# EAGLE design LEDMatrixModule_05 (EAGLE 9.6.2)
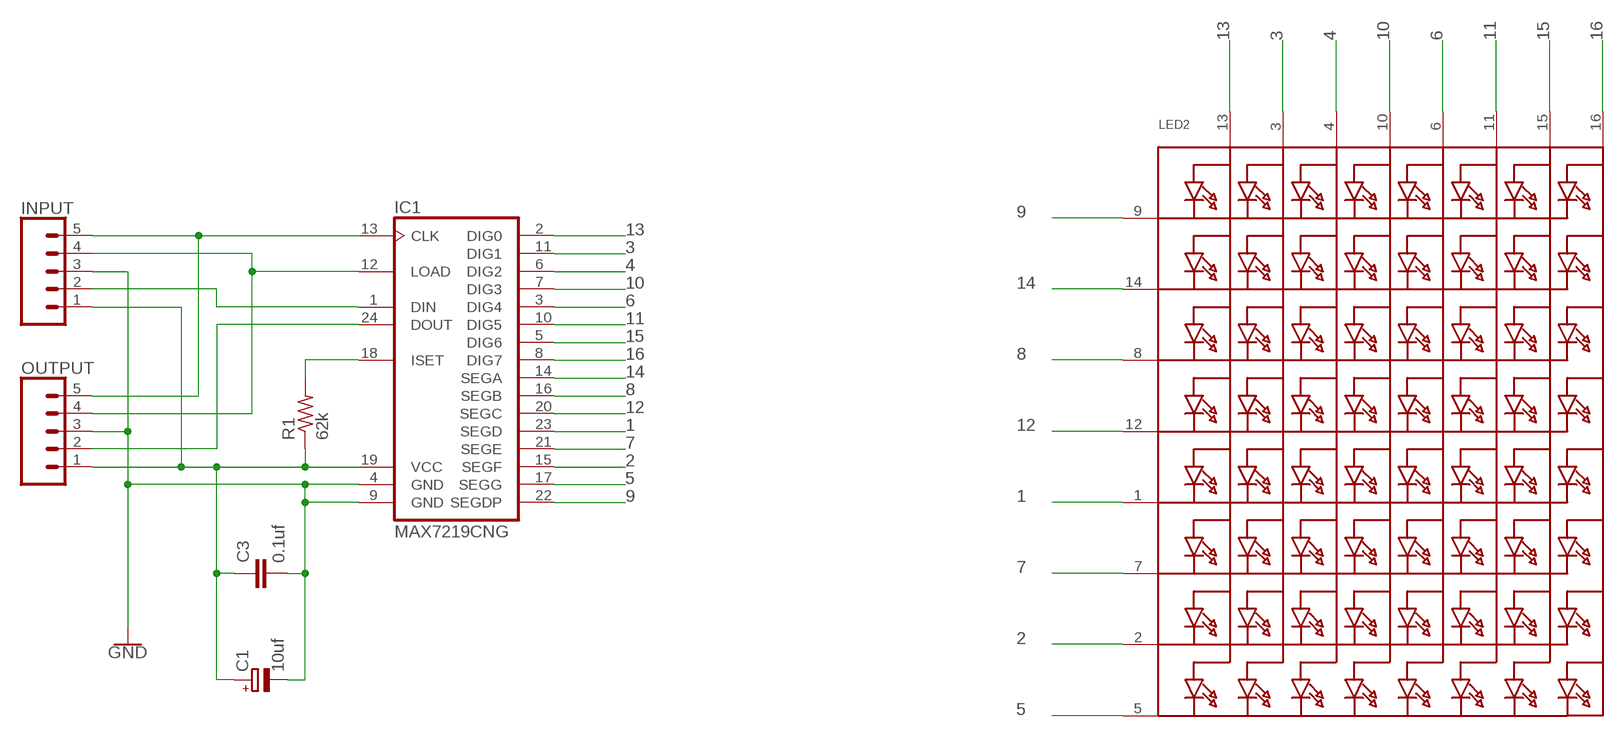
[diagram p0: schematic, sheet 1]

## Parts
C1  10uf  CPOL-EUE2.5-6  [E2,5-6]
C3  0.1uf  C2,5-3  [C2.5-3]
IC1  MAX7219CNG  [DIL24-3]
INPUT  CONN_05  [1X05]
LED2  SEGMENT_8X8_ROWCATHODEBL-M15  [SEGMENT_BL-M15A881]
OUTPUT  CONN_05  [1X05]
R1  62k  R-US_0309/10  [0309/10]

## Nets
1: IC1.23(SEGD) LED2.1(K5)
2: IC1.15(SEGF) LED2.2(K7)
3: IC1.11(DIG1) LED2.3(A2)
4: IC1.6(DIG2) LED2.4(A3)
5: IC1.17(SEGG) LED2.5(K8)
6: IC1.3(DIG4) LED2.6(A5)
7: IC1.21(SEGE) LED2.7(K6)
8: IC1.16(SEGB) LED2.8(K3)
9: IC1.22(SEGDP) LED2.9(K1)
10: IC1.7(DIG3) LED2.10(A4)
11: IC1.10(DIG5) LED2.11(A6)
12: IC1.20(SEGC) LED2.12(K4)
13: IC1.2(DIG0) LED2.13(A1)
14: IC1.14(SEGA) LED2.14(K2)
15: IC1.5(DIG6) LED2.15(A7)
16: IC1.8(DIG7) LED2.16(A8)
GND: C1.- C3.2 IC1.4(GND) IC1.9(GND) INPUT.3 OUTPUT.3
N$1: IC1.13(CLK) INPUT.5 OUTPUT.5
N$2: C1.+ C3.1 IC1.19(VCC) INPUT.1 OUTPUT.1 R1.1
N$3: IC1.18(ISET) R1.2
N$4: IC1.24(DOUT) OUTPUT.2
N$5: IC1.1(DIN) INPUT.2
N$6: IC1.12(LOAD) INPUT.4 OUTPUT.4

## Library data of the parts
C1 = rcl:CPOL-EU: POLARIZED CAPACITOR, European symbol
C3 = capacitor-wima:C: CAPACITOR
IC1 = max7219:MAX7219CNG: LED DISPLAY DRIVER; MF: MAXIM; MPN: MAX7219CNG; OC_FARNELL: 1523914; OC_NEWARK: 34C4018
INPUT OUTPUT = SparkFun-Connectors:CONN_05: Multi connection point. Often used as Generic Header-pin footprint for 0.1 inch spaced/style header connections On any of the 0.1 inch spaced packages, you can populate with these: Break Away Headers - Straight (PRT-00116) Break Away Male Headers - Right Angle (PRT-00553) Female Headers (PRT-00115)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
LED2 = adafruit:SEGMENT_8X8_ROWCATHODE: 8x8 LED Segment Displays: Row = Cathode 0.7" Red 8X8 Matrix, 1.9mm Round LEDs - BL-M07C881UR 1.2" Red 8x8 Matrix, 3.0mm Round LEDs - BL-M12A881UR 1.2" Red 8x8 Matrix, 3.0mm Square LEDs - BL-M12A883
R1 = BeagleBone_Black_Wireless:R-US_: RESISTOR, American symbol

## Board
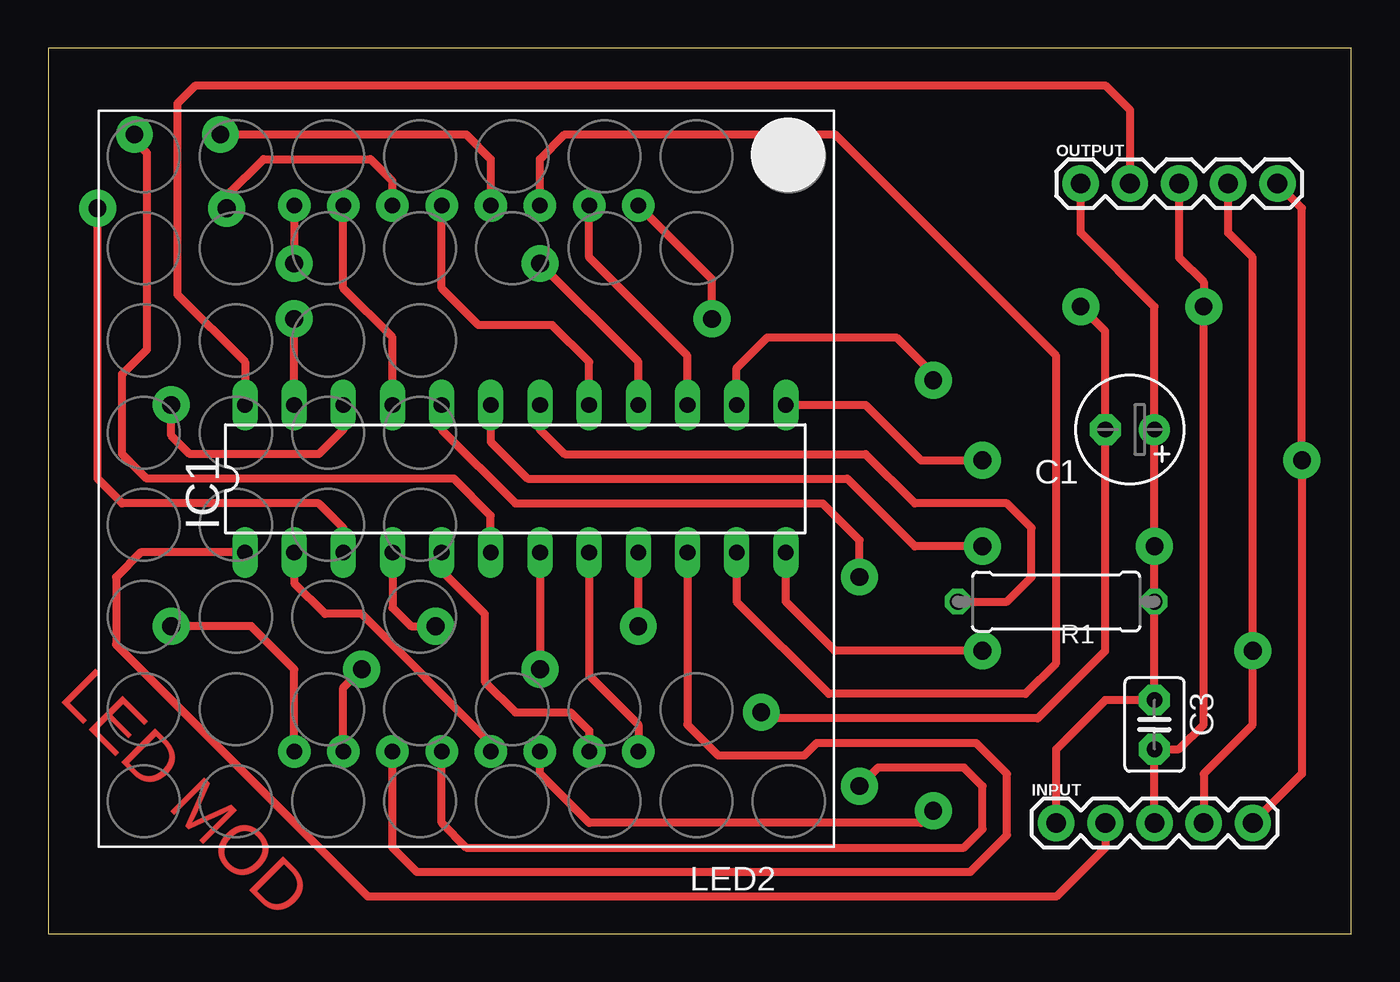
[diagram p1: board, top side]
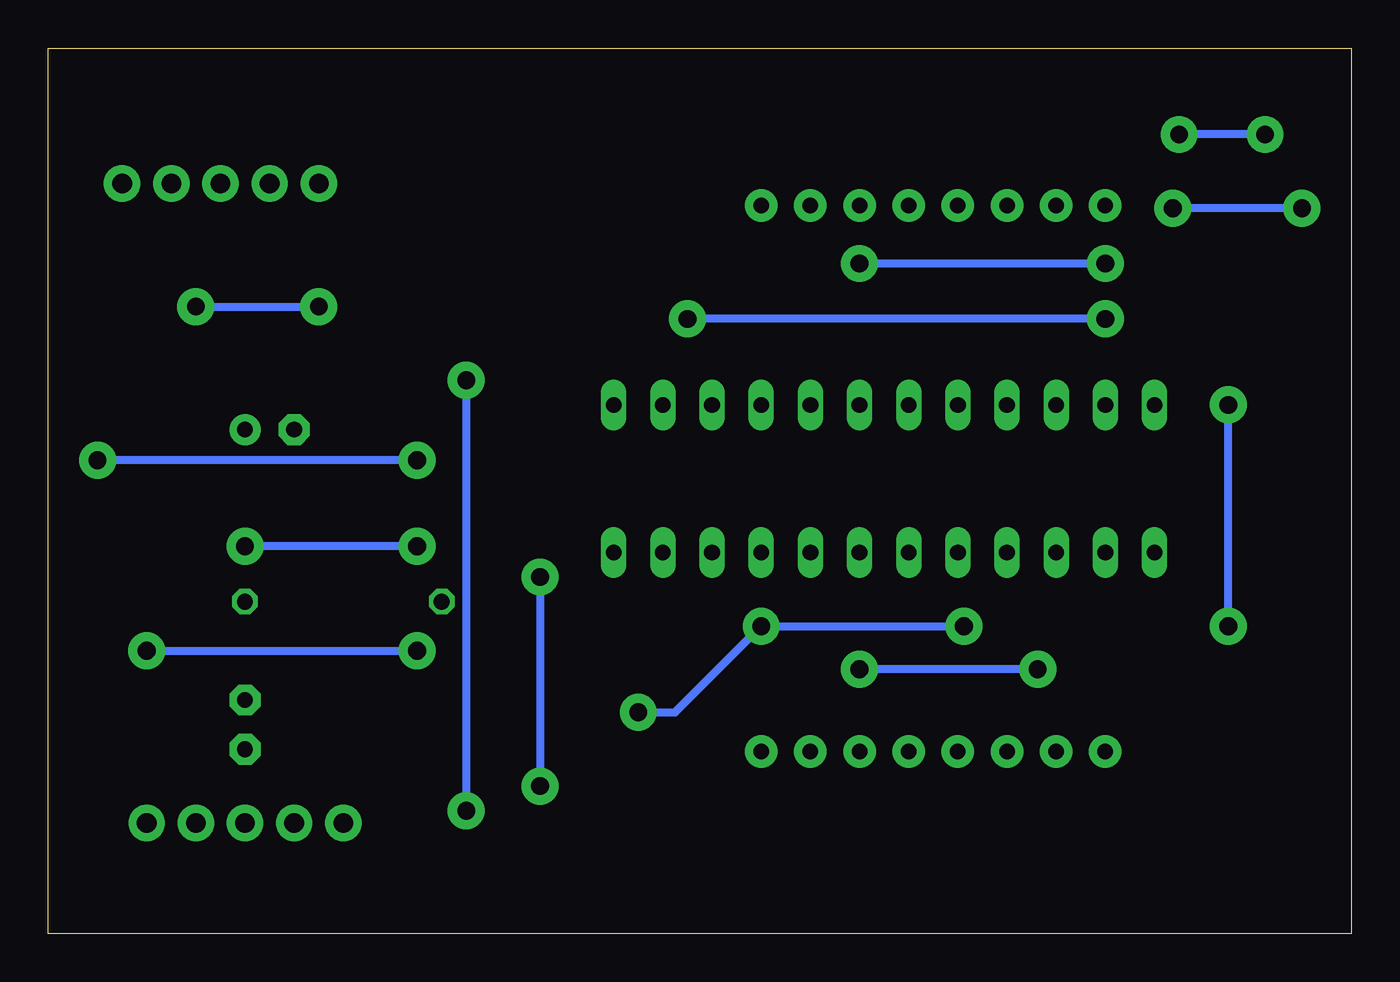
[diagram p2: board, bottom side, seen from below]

Size 67.31 x 45.72 mm. Coordinates in mm from the lower left corner, seen from the top.
Outline: 0,0 67.31,0 67.31,45.72 0,45.72 0,0
Copper layers (1*16): Top 0.035mm / dielectric 1.5mm / Bottom 0.035mm
Design rules "default": minimum track width 10mil, minimum drill 24mil, track to track 8mil, track to pad 8mil, pad to pad 8mil, via to via 8mil, smd to smd 8mil, copper to edge 40mil, drill to drill 8mil, minimum pad ring 10mil, minimum via ring 8mil, stop-mask expansion 4mil, vias tented up to drill 0mil, thermal gap 10mil

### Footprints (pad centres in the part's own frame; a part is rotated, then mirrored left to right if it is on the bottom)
E2,5-6 = drill 0.813 pad 1.6: + -1.27,0 | drill 0.813 pad 1.6 octagon: - 1.27,0
C2.5-3 = drill 0.813 pad 1.6 octagon: 1 -1.27,0; 2 1.27,0
DIL24-3 = drill 0.813 long: 1 -13.97,-3.81; 2 -11.43,-3.81; 3 -8.89,-3.81; 4 -6.35,-3.81; 5 -3.81,-3.81; 6 -1.27,-3.81; 7 1.27,-3.81; 8 3.81,-3.81; 9 6.35,-3.81; 10 8.89,-3.81; 11 11.43,-3.81; 12 13.97,-3.81; 13 13.97,3.81; 14 11.43,3.81; 15 8.89,3.81; 16 6.35,3.81; 17 3.81,3.81; 18 1.27,3.81; 19 -1.27,3.81; 20 -3.81,3.81; 21 -6.35,3.81; 22 -8.89,3.81; 23 -11.43,3.81; 24 -13.97,3.81
1X05 = drill 1.016 pad 1.88: 1 0,0; 2 2.54,0; 3 5.08,0; 4 7.62,0; 5 10.16,0
SEGMENT_BL-M15A881 = drill 0.8 pad 1.676: 1 -8.89,-14.1; 2 -6.35,-14.1; 3 -3.81,-14.1; 4 -1.27,-14.1; 5 1.27,-14.1; 6 3.81,-14.1; 7 6.35,-14.1; 8 8.89,-14.1; 9 8.89,14.1; 10 6.35,14.1; 11 3.81,14.1; 12 1.27,14.1; 13 -1.27,14.1; 14 -3.81,14.1; 15 -6.35,14.1; 16 -8.89,14.1
0309/10 = drill 0.813 octagon: 1 -5.08,0; 2 5.08,0

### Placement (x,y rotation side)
C1  55.88,26.04 180 top
C3  57.15,10.79 270 top
IC1  24.13,23.5 0 top
INPUT  52.07,5.71 0 top
LED2  21.59,23.5 180 top
OUTPUT  53.34,38.73 0 top
R1  52.07,17.14 180 top

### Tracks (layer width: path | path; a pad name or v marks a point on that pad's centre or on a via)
1  (via drill 0.91 pad 1.91)
  Top 0.406: IC1.23 v12.7,31.75 | v34.29,31.75 34.29,33.78 LED2.1
  Bottom 0.406: v12.7,31.75 v34.29,31.75
2
  Top 0.406: IC1.15 33.02,29.84 27.94,34.92 LED2.2
3
  Top 0.406: IC1.11 35.56,17.14 40.32,12.38 50.48,12.38 52.07,13.97 52.07,29.84 40.64,41.27 26.67,41.27 25.4,40.01 LED2.3
4  (via drill 0.91 pad 1.91)
  Top 0.406: v8.89,41.27 21.59,41.27 22.86,40.01 LED2.4 | v4.45,41.27 4.45,40.96 5.08,40.32 5.08,30.16 3.81,28.89 3.81,24.77 5.08,23.5 20.95,23.5 22.86,21.59 IC1.6
  Bottom 0.406: v4.45,41.27 v8.89,41.27
5
  Top 0.406: IC1.17 27.94,29.53 26.04,31.43 22.23,31.43 20.32,33.34 LED2.5
6  (via drill 0.91 pad 1.91)
  Top 0.406: IC1.3 15.24,20.95 13.97,22.23 3.81,22.23 2.54,23.5 v2.54,37.47 | LED2.6 17.78,38.87 16.64,40.01 11.11,40.01 9.21,38.1 v9.21,37.47
  Bottom 0.406: v2.54,37.47 v9.21,37.47
7
  Top 0.406: IC1.21 17.78,30.8 15.24,33.34 LED2.7
8  (via drill 0.91 pad 1.91)
  Top 0.406: IC1.16 30.48,29.53 v25.4,34.61 | LED2.8 v12.7,34.61
  Bottom 0.406: v12.7,34.61 v25.4,34.61
9  (via drill 0.91 pad 1.91)
  Top 0.406: IC1.22 15.24,26.04 13.97,24.77 7.3,24.77 6.35,25.72 v6.35,27.3 | LED2.9 12.7,13.65 10.48,15.88 v6.35,15.88
  Bottom 0.406: v6.35,15.88 v6.35,27.3
10  (via drill 0.91 pad 1.91)
  Top 0.406: IC1.7 v25.4,13.65 | LED2.10 15.24,12.7 v16.19,13.65
  Bottom 0.406: v16.19,13.65 v25.4,13.65
11
  Top 0.406: LED2.11 17.78,4.45 19.05,3.17 47.62,3.17 49.53,5.08 49.53,8.26 47.94,9.84 39.69,9.84 39.05,9.21 34.61,9.21 33.02,10.79 IC1.10
12  (via drill 0.91 pad 1.91)
  Top 0.406: LED2.12 20.32,5.71 21.59,4.45 47.31,4.45 48.26,5.4 48.26,7.62 47.31,8.57 42.86,8.57 v41.91,7.62 | IC1.20 20.32,26.04 24.13,22.23 40.01,22.23 41.91,20.32 v41.91,18.41
  Bottom 0.406: v41.91,18.41 v41.91,7.62
13
  Top 0.406: IC1.2 12.7,18.1 14.29,16.51 16.19,16.51 22.86,9.84 LED2.13
14  (via drill 0.91 pad 1.91)
  Top 0.406: LED2.14 25.4,8.26 27.94,5.71 45.09,5.71 v45.72,6.35 | IC1.14 35.56,29.21 37.15,30.8 43.81,30.8 45.72,28.89 v45.72,28.57
  Bottom 0.406: v45.72,28.57 v45.72,6.35
15
  Top 0.406: IC1.5 20.32,18.73 22.54,16.51 22.54,13.02 24.13,11.43 26.99,11.43 27.94,10.48 LED2.15
16
  Top 0.406: LED2.16 30.48,10.79 27.94,13.34 IC1.8
GND  (via drill 0.91 pad 1.91)
  Top 0.406: INPUT.3 C3.2 58.42,9.53 59.69,10.79 v59.69,32.38 59.69,33.66 58.42,34.92 OUTPUT.3 | v30.48,15.88 IC1.9 | v53.34,32.38 54.61,31.11 C1.- 54.61,14.61 51.12,11.11 37.15,11.11 v36.83,11.43 | IC1.4 17.78,16.83 18.73,15.88 v20,15.88
  Bottom 0.406: v20,15.88 v30.48,15.88 34.92,11.43 v36.83,11.43 | v59.69,32.38 v53.34,32.38
N$1  (via drill 0.91 pad 1.91)
  Top 0.406: IC1.13 42.23,27.3 45.09,24.45 v48.26,24.45 | INPUT.5 64.77,8.26 v64.77,24.45 64.77,37.47 OUTPUT.5
  Bottom 0.406: v48.26,24.45 v64.77,24.45
N$2  (via drill 0.91 pad 1.91)
  Top 0.406: INPUT.1 52.07,9.53 54.61,12.06 C3.1 R1.1 v57.15,20 C1.+ 57.15,32.38 53.34,36.2 OUTPUT.1 | v48.26,20 44.77,20 41.27,23.5 24.77,23.5 22.86,25.4 IC1.19
  Bottom 0.406: v48.26,20 v57.15,20
N$3
  Top 0.406: IC1.18 25.4,26.04 26.67,24.77 42.23,24.77 44.77,22.23 49.53,22.23 50.8,20.95 50.8,18.41 49.53,17.14 R1.2
N$4
  Top 0.406: OUTPUT.2 55.88,42.55 54.61,43.81 7.62,43.81 6.67,42.86 6.67,33.02 10.16,29.53 IC1.24
N$5
  Top 0.406: IC1.1 4.76,19.68 3.49,18.41 3.49,14.92 16.51,1.91 52.07,1.91 54.61,4.45 INPUT.2
N$6  (via drill 0.91 pad 1.91)
  Top 0.406: INPUT.4 59.69,8.26 62.23,10.79 v62.23,14.61 62.23,34.92 60.96,36.2 OUTPUT.4 | IC1.12 38.1,17.14 40.64,14.61 v48.26,14.61
  Bottom 0.406: v62.23,14.61 v48.26,14.61

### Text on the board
Top: LED MOD

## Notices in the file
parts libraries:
SparkFun-Connectors: Licensing: Creative Commons ShareAlike 4.0 International - https://creativecommons.org/licenses/by-sa/4.0
